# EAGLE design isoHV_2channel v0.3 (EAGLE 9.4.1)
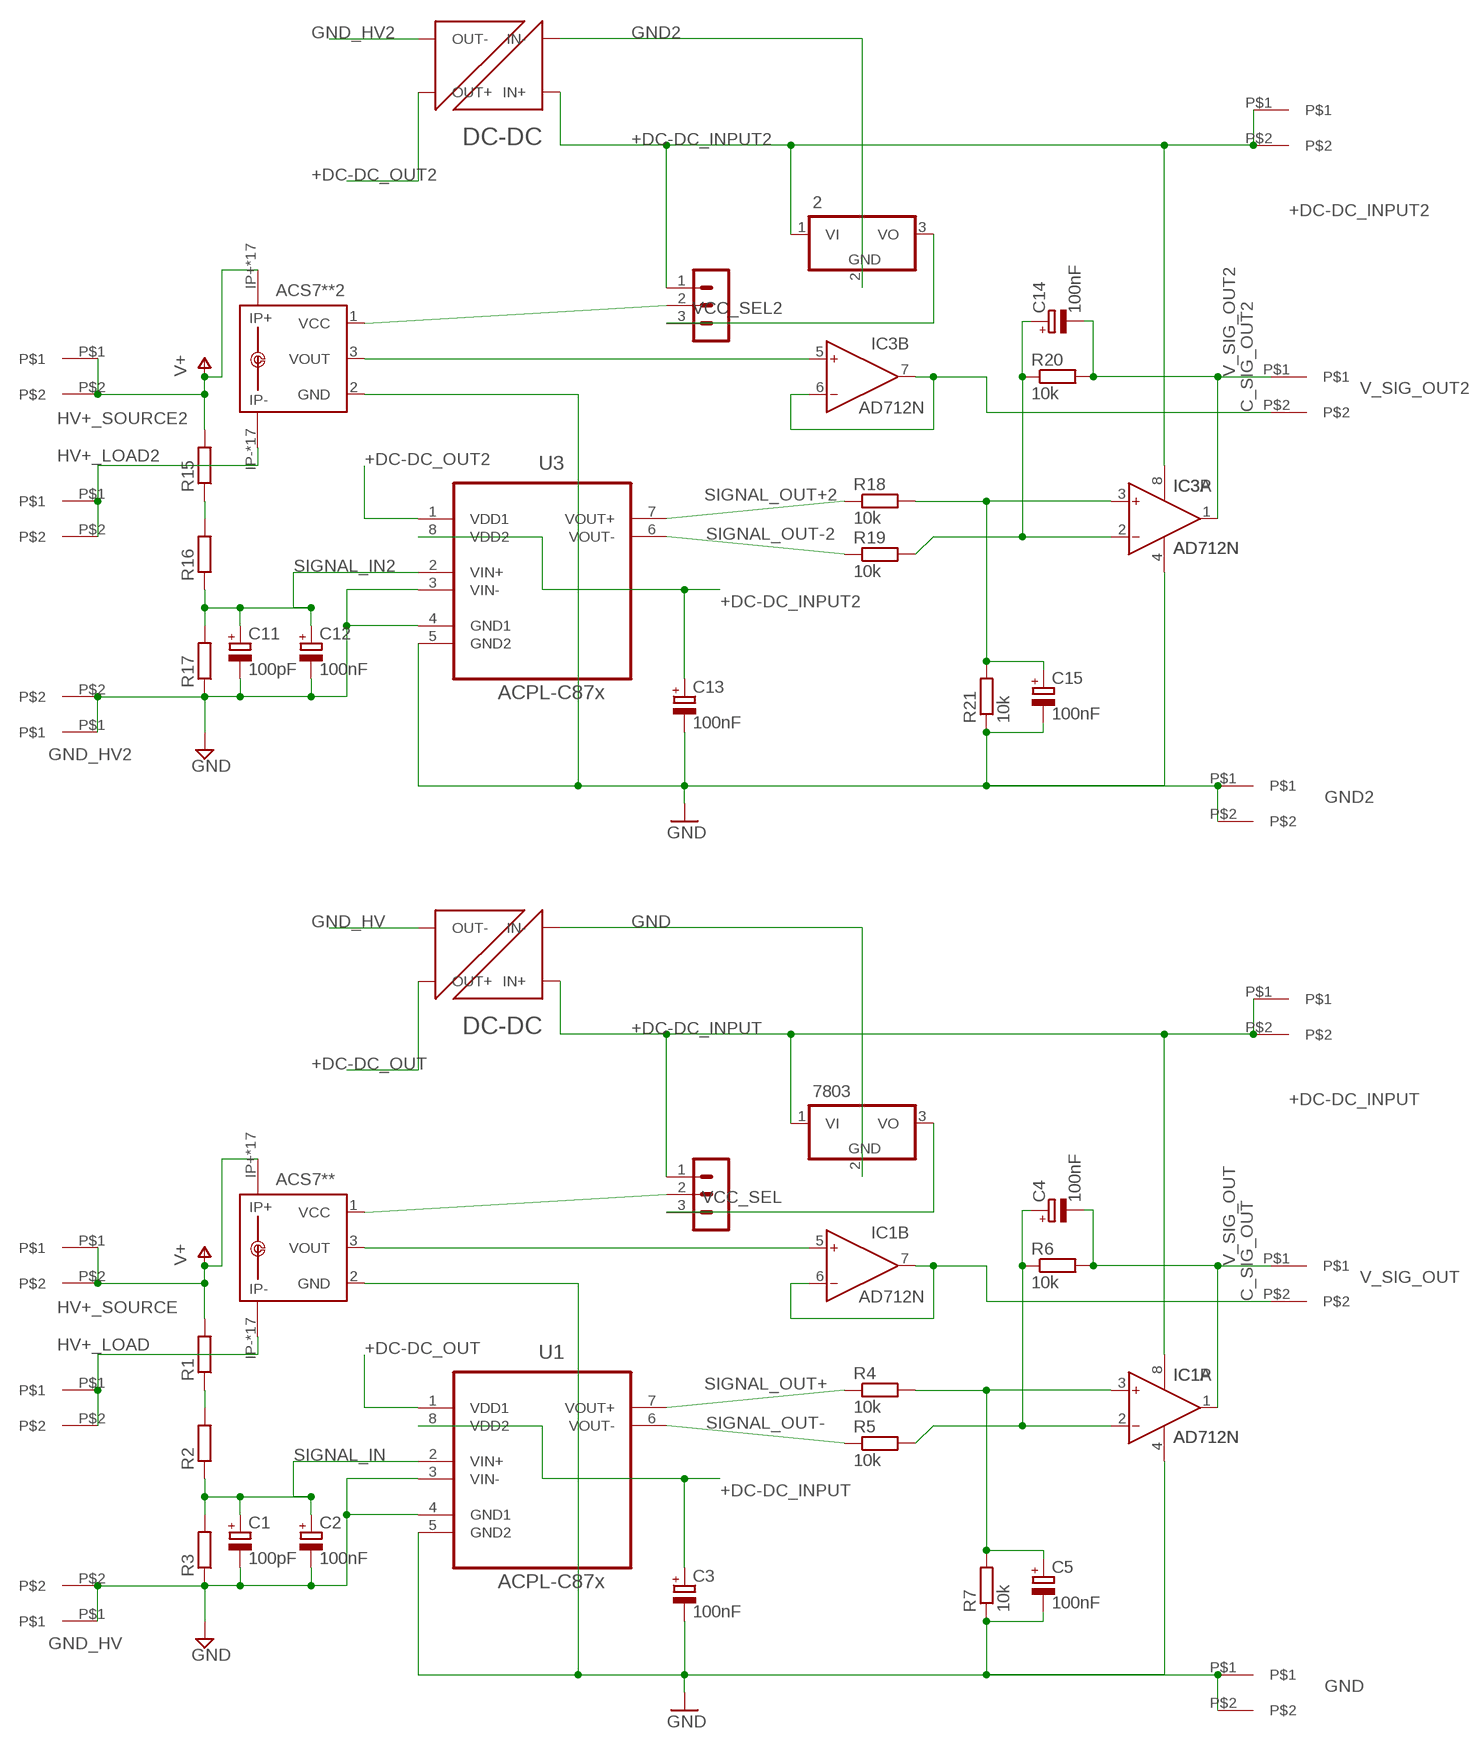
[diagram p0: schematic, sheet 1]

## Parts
2  7805TV  [TO220V]
7803  7805TV  [TO220V]
ACS7**  ACS758KCB-150B-PFF-T  [CB-PFF]
ACS7**2  ACS758KCB-150B-PFF-T  [CB-PFF]
C1  100pF  CPOL-EUB45181A  [B45181A]
C2  100nF  CPOL-EUB45181A  [B45181A]
C3  100nF  CPOL-EUB45181A  [B45181A]
C4  100nF  CPOL-EUB45181A  [B45181A]
C5  100nF  CPOL-EUB45181A  [B45181A]
C11  100pF  CPOL-EUB45181A  [B45181A]
C12  100nF  CPOL-EUB45181A  [B45181A]
C13  100nF  CPOL-EUB45181A  [B45181A]
C14  100nF  CPOL-EUB45181A  [B45181A]
C15  100nF  CPOL-EUB45181A  [B45181A]
IC1  AD712N  [DIL08]
IC3  AD712N  [DIL08]
R1  R-EU_0411/15  [0411/15]
R2  R-EU_0411/15  [0411/15]
R3  R-EU_0411/15  [0411/15]
R4  10k  R-EU_0204/7  [0204/7]
R5  10k  R-EU_0204/7  [0204/7]
R6  10k  R-EU_0204/7  [0204/7]
R7  10k  R-EU_0204/7  [0204/7]
R15  R-EU_0411/15  [0411/15]
R16  R-EU_0411/15  [0411/15]
R17  R-EU_0411/15  [0411/15]
R18  10k  R-EU_0204/7  [0204/7]
R19  10k  R-EU_0204/7  [0204/7]
R20  10k  R-EU_0204/7  [0204/7]
R21  10k  R-EU_0204/7  [0204/7]
U1  ACPL-C87x  ACPL-C79B-000E  [SOIC127P1150X330-8N]
U3  ACPL-C87x  ACPL-C79B-000E  [SOIC127P1150X330-8N]
U$1  7.62MM_TERMINAL_BLOCK  [7.62MM]
U$2  7.62MM_TERMINAL_BLOCK  [7.62MM]
U$3  7.62MM_TERMINAL_BLOCK  [7.62MM]
U$4  7.62MM_TERMINAL_BLOCK  [7.62MM]
U$5  7.62MM_TERMINAL_BLOCK  [7.62MM]
U$6  7.62MM_TERMINAL_BLOCK  [7.62MM]
U$7  NXF1  [NXF1]
U$15  7.62MM_TERMINAL_BLOCK  [7.62MM]
U$16  7.62MM_TERMINAL_BLOCK  [7.62MM]
U$17  7.62MM_TERMINAL_BLOCK  [7.62MM]
U$18  7.62MM_TERMINAL_BLOCK  [7.62MM]
U$19  7.62MM_TERMINAL_BLOCK  [7.62MM]
U$20  7.62MM_TERMINAL_BLOCK  [7.62MM]
U$21  NXF1  [NXF1]
VCC_SEL  MA03-1  [MA03-1]
VCC_SEL2  MA03-1  [MA03-1]

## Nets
+DC-DC_INPUT: 7803.1(VI) C3.+ IC1.8(P:V+) U1.8(VDD2) U$3.P$1 U$3.P$2 U$7.P$3(IN+) VCC_SEL.1
+DC-DC_INPUT2: 2.1(VI) C13.+ IC3.8(P:V+) U3.8(VDD2) U$17.P$1 U$17.P$2 U$21.P$3(IN+) VCC_SEL2.1
+DC-DC_OUT: U1.1(VDD1) U$7.P$8(OUT+)
+DC-DC_OUT2: U3.1(VDD1) U$21.P$8(OUT+)
C_SIG_OUT: IC1.6(B:IN-) IC1.7(B:OUT) U$5.P$2
C_SIG_OUT2: IC3.6(B:IN-) IC3.7(B:OUT) U$19.P$2
GND: 7803.2(GND) ACS7**.2(GND) C3.- C5.- IC1.4(P:V-) R7.1 U1.5(GND2) U$4.P$1 U$4.P$2 U$7.P$1(IN-)
GND2: 2.2(GND) ACS7**2.2(GND) C13.- C15.- IC3.4(P:V-) R21.1 U3.5(GND2) U$18.P$1 U$18.P$2 U$21.P$1(IN-) ; supply symbol labelled GND
GND_HV: C1.- C2.- R3.1 U1.3(VIN-) U1.4(GND1) U$2.P$1 U$2.P$2 U$7.P$7(OUT-) ; supply symbol labelled GND
GND_HV2: C11.- C12.- R17.1 U3.3(VIN-) U3.4(GND1) U$16.P$1 U$16.P$2 U$21.P$7(OUT-) ; supply symbol labelled GND
HV+_LOAD: ACS7**.IP- ACS7**.IP-@2(IP-) ACS7**.IP-@3(IP-) ACS7**.IP-@4(IP-) ACS7**.IP-@5(IP-) ACS7**.IP-@6(IP-) ACS7**.IP-@7(IP-) ACS7**.IP-@8(IP-) ACS7**.IP-@9(IP-) ACS7**.IP-@10(IP-) ACS7**.IP-@11(IP-) ACS7**.IP-@12(IP-) ACS7**.IP-@13(IP-) ACS7**.IP-@14(IP-) ACS7**.IP-@15(IP-) ACS7**.IP-@16(IP-) ACS7**.IP-@17(IP-) U$6.P$1 U$6.P$2
HV+_LOAD2: ACS7**2.IP- ACS7**2.IP-@2(IP-) ACS7**2.IP-@3(IP-) ACS7**2.IP-@4(IP-) ACS7**2.IP-@5(IP-) ACS7**2.IP-@6(IP-) ACS7**2.IP-@7(IP-) ACS7**2.IP-@8(IP-) ACS7**2.IP-@9(IP-) ACS7**2.IP-@10(IP-) ACS7**2.IP-@11(IP-) ACS7**2.IP-@12(IP-) ACS7**2.IP-@13(IP-) ACS7**2.IP-@14(IP-) ACS7**2.IP-@15(IP-) ACS7**2.IP-@16(IP-) ACS7**2.IP-@17(IP-) U$20.P$1 U$20.P$2
HV+_SOURCE: ACS7**.IP+ ACS7**.IP+@2(IP+) ACS7**.IP+@3(IP+) ACS7**.IP+@4(IP+) ACS7**.IP+@5(IP+) ACS7**.IP+@6(IP+) ACS7**.IP+@7(IP+) ACS7**.IP+@8(IP+) ACS7**.IP+@9(IP+) ACS7**.IP+@10(IP+) ACS7**.IP+@11(IP+) ACS7**.IP+@12(IP+) ACS7**.IP+@13(IP+) ACS7**.IP+@14(IP+) ACS7**.IP+@15(IP+) ACS7**.IP+@16(IP+) ACS7**.IP+@17(IP+) R1.2 U$1.P$1 U$1.P$2 ; supply symbol labelled V+
HV+_SOURCE2: ACS7**2.IP+ ACS7**2.IP+@2(IP+) ACS7**2.IP+@3(IP+) ACS7**2.IP+@4(IP+) ACS7**2.IP+@5(IP+) ACS7**2.IP+@6(IP+) ACS7**2.IP+@7(IP+) ACS7**2.IP+@8(IP+) ACS7**2.IP+@9(IP+) ACS7**2.IP+@10(IP+) ACS7**2.IP+@11(IP+) ACS7**2.IP+@12(IP+) ACS7**2.IP+@13(IP+) ACS7**2.IP+@14(IP+) ACS7**2.IP+@15(IP+) ACS7**2.IP+@16(IP+) ACS7**2.IP+@17(IP+) R15.2 U$15.P$1 U$15.P$2 ; supply symbol labelled V+
N$1: C5.+ IC1.3(A:IN+) R4.2 R7.2
N$2: R1.1 R2.2
N$3: ACS7**.1(VCC) VCC_SEL.2
N$5: C4.+ IC1.2(A:IN-) R5.2 R6.1
N$6: ACS7**.3(VOUT) IC1.5(B:IN+)
N$7: 7803.3(VO) VCC_SEL.3
N$132: R15.1 R16.2
N$142: C15.+ IC3.3(A:IN+) R18.2 R21.2
N$152: C14.+ IC3.2(A:IN-) R19.2 R20.1
N$162: ACS7**2.1(VCC) VCC_SEL2.2
N$172: ACS7**2.3(VOUT) IC3.5(B:IN+)
N$182: 2.3(VO) VCC_SEL2.3
SIGNAL_IN: C1.+ C2.+ R2.1 R3.2 U1.2(VIN+)
SIGNAL_IN2: C11.+ C12.+ R16.1 R17.2 U3.2(VIN+)
SIGNAL_OUT+: R4.1 U1.7(VOUT+)
SIGNAL_OUT+2: R18.1 U3.7(VOUT+)
SIGNAL_OUT-: R5.1 U1.6(VOUT-)
SIGNAL_OUT-2: R19.1 U3.6(VOUT-)
V_SIG_OUT: C4.- IC1.1(A:OUT) R6.2 U$5.P$1
V_SIG_OUT2: C14.- IC3.1(A:OUT) R20.2 U$19.P$1

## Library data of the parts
2 7803 = linear:78*: Positive VOLTAGE REGULATOR Source: http://cache.national.com/ds/LM/LM78L05.pdf http://www.fairchildsemi.com/ds/LM/LM7805.pdf
ACS7** ACS7**2 = allegro:ACS758*: Thermally Enhanced, Fully Integrated, Hall Effect-Based Linear Current Sensor with 100 micro Ohm Current Conductor display layer 49 Reference in BRD and place VIAs on circles Source: http://www.allegromicro.com/en/Products/Part_Numbers/0758/0758.pdf; MPN: ACS7**; OC_FARNELL: 1718995; OC_NEWARK: 04R7129
C1-C5 C11-C15 = rcl:CPOL-EU: POLARIZED CAPACITOR, European symbol; SPICEPREFIX: C
IC1 IC3 = analog-devices:AD712: Dual Precision, Low Cost, High Speed BiFET Op Amp Source: http://www.analog.com/static/imported-files/data_sheets/AD712.pdf; MF: ALTERA CORPORATION; MPN: AD712JNZ; OC_FARNELL: 9604898; OC_NEWARK: 59K4554
R1-R7 R15-R21 = rcl:R-EU_: RESISTOR, European symbol; SPICEPREFIX: R
U1 U3 = Avago_By_element14_Batch_1:ACPL-C79B-000E: Precision Miniature Isolation Amplifiers; DESCRIPTION: Precision Miniature Isolation Amplifiers; MPN: ACPL-C79B-000E; OC_FARNELL: 1854253; OC_NEWARK: 74R5803; PACKAGE: SOIC-8; SUPPLIER: AVAGO TECHNOLOGIES
U$1-U$6 U$15-U$20 = 7.62mm terminal block:7.62MM_TERMINAL_BLOCK
U$7 U$21 = NXF1:NXF1
VCC_SEL VCC_SEL2 = con-lstb:MA03-1: PIN HEADER; OC_FARNELL: unknown; OC_NEWARK: unknown

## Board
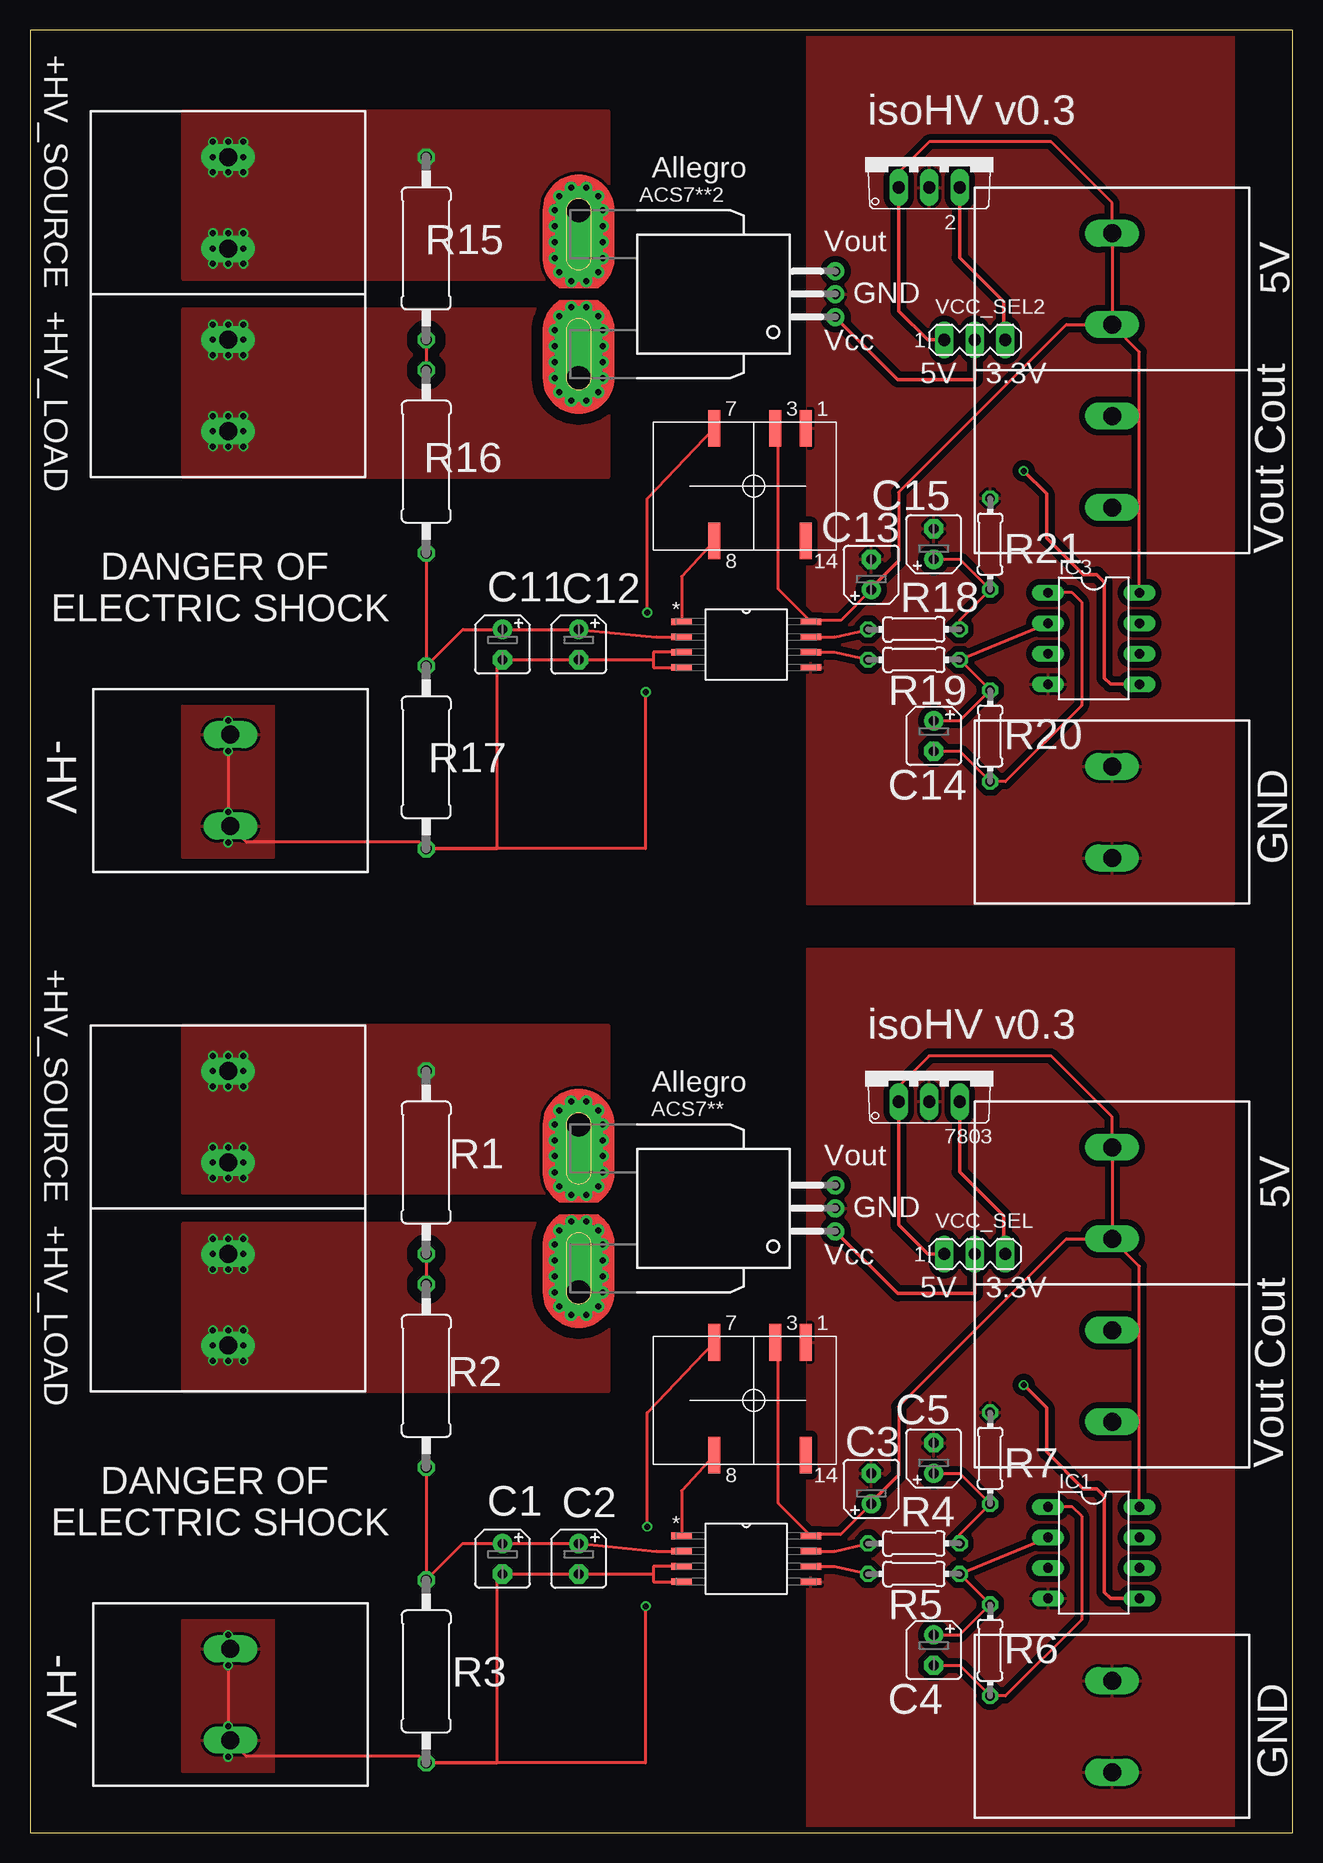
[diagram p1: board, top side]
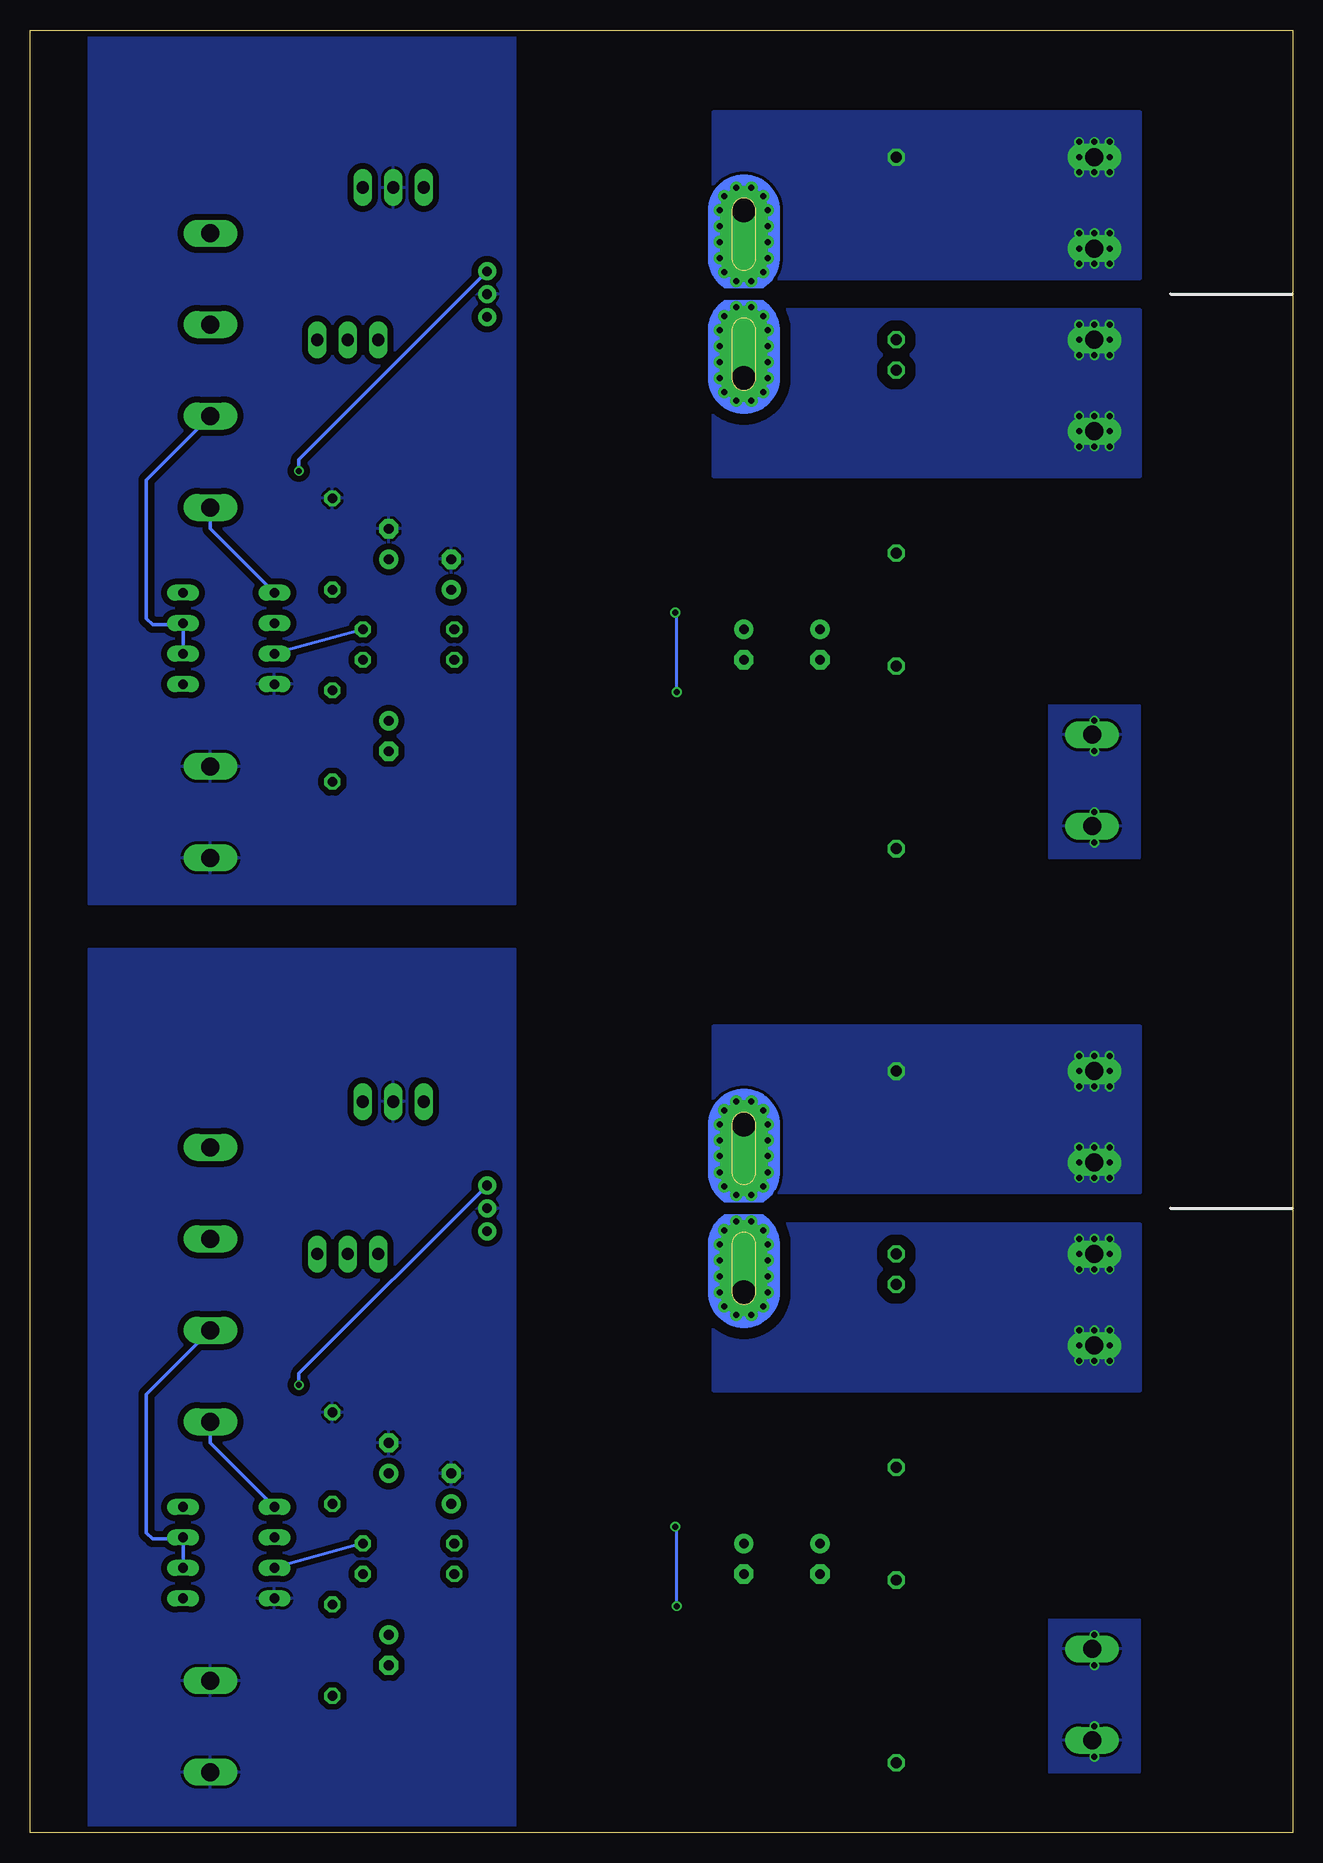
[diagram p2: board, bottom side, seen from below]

Size 105.21 x 150.29 mm. Coordinates in mm from the lower left corner, seen from the top.
Outline: 0,150.29 0,0 105.21,0 105.21,150.29 0,150.29
Copper layers (1*16): Top 0.07111875mm / dielectric 1.45776875mm / Bottom 0.07111875mm
Design rules "jlcpcb *": minimum track width 6mil, minimum drill 12mil, track to track 10mil, track to pad 10mil, pad to pad 10mil, via to via 10mil, smd to smd 0mil, copper to edge 10mil, drill to drill 10mil, minimum pad ring 10mil, minimum via ring 6mil, stop-mask expansion 2mil, vias tented up to drill 25mil, thermal gap 10mil

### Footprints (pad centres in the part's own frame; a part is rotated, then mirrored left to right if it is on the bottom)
TO220V = drill 1.016 long: 1 -2.54,-2.54; 2 0,-2.54; 3 2.54,-2.54
CB-PFF = drill 0.8 pad 1.5: 1 -1.91,-21.4; 2 0,-21.4; 3 1.91,-21.4 | drill 2 pad 4 offset: IP+ 7,0; IP- -7,0 | drill 0.5 pad 0.9: IP+@2 8.89,0.635; IP+@3 8.89,-0.635; IP+@4 8.175,-1.625; IP+@5 7,-2; IP+@6 5.675,-2; IP+@7 4.35,-2; IP+@8 3,-2; IP+@9 1.825,-1.625; IP+@10 1.1,-0.625; IP+@11 1.1,0.625; IP+@12 1.825,1.625; IP+@13 3,2; IP+@14 4.35,2; IP+@15 5.675,2; IP+@16 7,2; IP+@17 8.175,1.625; IP-@2 -8.89,0.635; IP-@3 -8.89,-0.635; IP-@4 -8.175,-1.625; IP-@5 -7,-2; IP-@6 -5.675,-2; IP-@7 -4.325,-2; IP-@8 -3,-2; IP-@9 -1.825,-1.625; IP-@10 -1.1,-0.625; IP-@11 -1.1,0.625; IP-@12 -1.825,1.625; IP-@13 -3,2; IP-@14 -4.325,2; IP-@15 -5.675,2; IP-@16 -7,2; IP-@17 -8.175,1.625
B45181A = drill 0.813 pad 1.6: + -1.27,0 | drill 0.813 pad 1.6 octagon: - 1.27,0
DIL08 = drill 0.813 long: 1 -3.81,-3.81; 2 -1.27,-3.81; 3 1.27,-3.81; 4 3.81,-3.81; 5 3.81,3.81; 6 1.27,3.81; 7 -1.27,3.81; 8 -3.81,3.81
0411/15 = drill 0.914 octagon: 1 -7.62,0; 2 7.62,0
0204/7 = drill 0.813 octagon: 1 -3.81,0; 2 3.81,0
SOIC127P1150X330-8N = smd 1.702 x 0.559: 1 -5.385,1.905; 2 -5.385,0.635; 3 -5.385,-0.635; 4 -5.385,-1.905; 5 5.385,-1.905; 6 5.385,-0.635; 7 5.385,0.635; 8 5.385,1.905
7.62MM = drill 1.5 long: P$1 0,-3.81; P$2 0,3.81
NXF1 = smd 0.991 x 3.048: P$1 -4.318,-4.826; P$3 -1.778,-4.826; P$7 3.302,-4.826; P$8 3.302,4.572; P$14 -4.318,4.572
MA03-1 = drill 1.016 long: 1 -2.54,0; 2 0,0; 3 2.54,0

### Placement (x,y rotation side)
2  74.93,139.7 0 top
7803  74.93,63.5 0 top
ACS7**  45.72,52.07 90 top
ACS7**2  45.72,128.27 90 top
C1  39.37,22.86 270 top
C2  45.72,22.86 270 top
C3  70.1,28.7 90 top
C4  75.31,15.24 270 top
C5  75.31,31.24 90 top
C11  39.37,99.06 270 top
C12  45.72,99.06 270 top
C13  70.1,104.9 90 top
C14  75.31,91.44 270 top
C15  75.31,107.44 90 top
IC1  88.65,23.37 270 top
IC3  88.65,99.57 270 top
R1  33.02,55.88 90 top
R2  33.02,38.1 90 top
R3  33.02,13.46 90 top
R4  73.66,24.13 0 top
R5  73.66,21.59 0 top
R6  80.01,15.24 270 top
R7  80.01,31.24 270 top
R15  33.02,132.08 90 top
R16  33.02,114.3 90 top
R17  33.02,89.66 90 top
R18  73.66,100.33 0 top
R19  73.66,97.79 0 top
R20  80.01,91.44 270 top
R21  80.01,107.44 270 top
U1  59.69,22.86 0 top
U3  59.69,99.06 0 top
U$1  16.51,59.69 180 top
U$2  16.7,11.54 0 top
U$3  90.17,53.34 0 top
U$4  90.17,8.89 180 top
U$5  90.17,38.1 0 top
U$6  16.51,44.45 0 top
U$7  60.33,36.07 180 top
U$15  16.51,135.89 180 top
U$16  16.7,87.74 0 top
U$17  90.17,129.54 0 top
U$18  90.17,85.09 180 top
U$19  90.17,114.3 0 top
U$20  16.51,120.65 0 top
U$21  60.33,112.27 180 top
VCC_SEL  78.74,48.26 0 top
VCC_SEL2  78.74,124.46 0 top

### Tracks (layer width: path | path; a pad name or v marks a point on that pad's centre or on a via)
+DC-DC_INPUT
  Top 0.254: IC1.8 92.46,47.24 U$3.P$1 | U$3.P$1 U$3.P$2 90.17,59.69 85.09,64.77 74.93,64.77 72.39,62.23 7803.1 | 72.39,30.73 72.39,35.56 86.36,49.53 U$3.P$1 | C3.+ 67.55,24.88 65.08,24.88 U1.8 62.36,27.48 62.36,40.59 U$7.P$3
  Top 0.305: 7803.1 72.39,50.67 74.8,48.26 VCC_SEL.1 | 72.39,30.73 72.39,29.84 70.1,27.56 C3.+
+DC-DC_INPUT2
  Top 0.254: IC3.8 92.46,123.44 U$17.P$1 | U$17.P$1 U$17.P$2 90.17,135.89 85.09,140.97 74.93,140.97 72.39,138.43 2.1 | 72.39,106.93 72.39,111.76 86.36,125.73 U$17.P$1 | C13.+ 67.55,101.08 65.08,101.08 U3.8 62.36,103.68 62.36,116.79 U$21.P$3
  Top 0.305: 2.1 72.39,126.87 74.8,124.46 VCC_SEL2.1 | 72.39,106.93 72.39,106.05 70.1,103.76 C13.+
+DC-DC_OUT
  Top 0.254: U1.1 54.3,28.54 U$7.P$8
+DC-DC_OUT2
  Top 0.254: U3.1 54.3,104.74 U$21.P$8
C_SIG_OUT
  Bottom 0.305: U$5.P$2 95.5,36.58 95.5,25.02 95,24.51 92.58,24.51 IC1.7 IC1.6
C_SIG_OUT2
  Bottom 0.305: U$19.P$2 95.5,112.78 95.5,101.22 95,100.71 92.58,100.71 IC3.7 IC3.6
GND
  pour Bottom (isolate 0.508): 100.33,73.66 100.33,0 64.77,0 64.77,73.66
  pour Top (isolate 0.508): 64.77,73.66 64.77,0 100.33,0 100.33,73.66
GND2
  pour Bottom (isolate 0.508): 100.33,149.86 100.33,77.47 64.77,77.47 64.77,149.86
  pour Top (isolate 0.508): 64.77,151.13 64.77,77.47 100.33,77.47 100.33,151.13
GND_HV  (via drill 0.5)
  Top 0.254: U1.3 51.94,22.23 51.94,21.59 | 51.94,21.59 51.94,20.95 U1.4 | U$2.P$2 16.7,14.16 v16.51,13.97 v16.51,8.89 16.7,8.7 U$2.P$1 18.04,6.39 32.47,6.39 R3.1 | R3.1 38.9,5.84 38.9,21.12 C1.- C2.- 51.94,21.59 | R3.1 51.31,5.84 v51.31,18.9 | v51.44,25.53 51.44,35.02 U$7.P$7
  Bottom 0.254: v51.31,18.9 51.31,25.4 v51.44,25.53
  other vias: 16.51,16.51 16.51,6.35
  pour Top: 12.7,17.78 20.32,17.78 20.32,5.08 12.7,5.08
  pour Bottom: 12.7,17.78 20.32,17.78 20.32,5.08 12.7,5.08
GND_HV2  (via drill 0.5)
  Top 0.254: U3.3 51.94,98.42 51.94,97.79 | 51.94,97.79 51.94,97.16 U3.4 | U$16.P$2 16.7,90.36 v16.51,90.17 v16.51,85.09 16.7,84.9 U$16.P$1 18.04,82.59 32.47,82.59 R17.1 | R17.1 38.9,82.04 38.9,97.32 C11.- C12.- 51.94,97.79 | R17.1 51.31,82.04 v51.31,95.1 | v51.44,101.73 51.44,111.22 U$21.P$7
  Bottom 0.254: v51.31,95.1 51.31,101.6 v51.44,101.73
  other vias: 16.51,92.71 16.51,82.55
  pour Top: 12.7,93.98 20.32,93.98 20.32,81.28 12.7,81.28
  pour Bottom: 12.7,93.98 20.32,93.98 20.32,81.28 12.7,81.28
HV+_LOAD  (via drill 0.5)
  other vias: 16.51,46.99 15.24,49.53 16.51,49.53 17.78,49.53 17.78,48.26 17.78,46.99 15.24,46.99 15.24,48.26 17.78,41.91 17.78,40.64 17.78,39.37 16.51,39.37 15.24,39.37 15.24,40.64 15.24,41.91 16.51,41.91
  pour Bottom (isolate 0.889, no thermals): 48.26,50.8 12.7,50.8 12.7,36.83 48.26,36.83
  pour Top (isolate 0.889, no thermals): 48.26,50.8 12.7,50.8 12.7,36.83 48.26,36.83
HV+_LOAD2  (via drill 0.5)
  other vias: 16.51,123.19 15.24,125.73 16.51,125.73 17.78,125.73 17.78,124.46 17.78,123.19 15.24,123.19 15.24,124.46 17.78,118.11 17.78,116.84 17.78,115.57 16.51,115.57 15.24,115.57 15.24,116.84 15.24,118.11 16.51,118.11
  pour Bottom (isolate 0.889, no thermals): 48.26,127 12.7,127 12.7,113.03 48.26,113.03
  pour Top (isolate 0.889, no thermals): 48.26,127 12.7,127 12.7,113.03 48.26,113.03
HV+_SOURCE  (via drill 0.5)
  other vias: 15.24,57.15 16.51,57.15 17.78,57.15 17.78,55.88 17.78,54.61 16.51,54.61 15.24,54.61 15.24,55.88 16.51,62.23 17.78,62.23 17.78,63.5 17.78,64.77 16.51,64.77 15.24,64.77 15.24,63.5 15.24,62.23
  pour Top (no thermals): 46.99,48.26 48.26,49.53 48.26,48.26
  pour Bottom (no thermals): 12.7,53.34 48.26,53.34 48.26,67.31 12.7,67.31
  pour Top (no thermals): 12.7,53.34 48.26,53.34 48.26,67.31 12.7,67.31
HV+_SOURCE2  (via drill 0.5)
  other vias: 15.24,133.35 16.51,133.35 17.78,133.35 17.78,132.08 17.78,130.81 16.51,130.81 15.24,130.81 15.24,132.08 16.51,138.43 17.78,138.43 17.78,139.7 17.78,140.97 16.51,140.97 15.24,140.97 15.24,139.7 15.24,138.43
  pour Top (no thermals): 46.99,124.46 48.26,125.73 48.26,124.46
  pour Bottom (no thermals): 12.7,129.54 48.26,129.54 48.26,143.51 12.7,143.51
  pour Top (no thermals): 12.7,129.54 48.26,129.54 48.26,143.51 12.7,143.51
N$1
  Top 0.254: R4.2 77.47,24.89 R7.2 77.47,29.97 C5.+
  Bottom 0.254: R4.2 IC1.3
N$2
  Top 0.254: R1.1 R2.2
N$3
  Top 0.305: VCC_SEL.2 78.74,44.96 72.32,44.96 ACS7**.1
N$5
  Top 0.254: IC1.2 R5.2 R6.1 77.47,16.51 C4.+
N$6  (via drill 0.5)
  Top 0.305: v82.8,37.34 84.71,35.43 84.71,31.75 87.76,28.7 88.9,28.7 89.53,28.07 89.53,20.07 90.04,19.56 IC1.5
  Bottom 0.305: v82.8,37.34 82.8,38.3 ACS7**.3
N$7
  Top 0.305: 7803.3 77.47,55.12 81.15,51.44 81.15,48.39 VCC_SEL.3
N$132
  Top 0.254: R15.1 R16.2
N$142
  Top 0.254: R18.2 77.47,101.09 R21.2 77.47,106.17 C15.+
  Bottom 0.254: R18.2 IC3.3
N$152
  Top 0.254: IC3.2 R19.2 R20.1 77.47,92.71 C14.+
N$162
  Top 0.305: VCC_SEL2.2 78.74,121.16 72.32,121.16 ACS7**2.1
N$172  (via drill 0.5)
  Top 0.305: v82.8,113.54 84.71,111.63 84.71,107.95 87.76,104.9 88.9,104.9 89.53,104.27 89.53,96.27 90.04,95.76 IC3.5
  Bottom 0.305: v82.8,113.54 82.8,114.5 ACS7**2.3
N$182
  Top 0.305: 2.3 77.47,131.32 81.15,127.64 81.15,124.59 VCC_SEL2.3
SIGNAL_IN
  Top 0.254: R2.1 R3.2 36.07,24.13 C1.+ C2.+ 52.2,23.5 U1.2
SIGNAL_IN2
  Top 0.254: R16.1 R17.2 36.07,100.33 C11.+ C12.+ 52.2,99.69 U3.2
SIGNAL_OUT+
  Top 0.254: U1.7 67.06,23.5 R4.1
SIGNAL_OUT+2
  Top 0.254: U3.7 67.06,99.69 R18.1
SIGNAL_OUT-
  Top 0.254: U1.6 67.06,22.23 R5.1
SIGNAL_OUT-2
  Top 0.254: U3.6 67.06,98.42 R19.1
V_SIG_OUT
  Top 0.254: C4.- 77.47,13.97 R6.2 81.28,11.43 87.63,17.78 87.63,26.42 86.87,27.18 IC1.1
  Bottom 0.305: U$5.P$1 90.17,32.51 IC1.1
V_SIG_OUT2
  Top 0.254: C14.- 77.47,90.17 R20.2 81.28,87.63 87.63,93.98 87.63,102.62 86.87,103.38 IC3.1
  Bottom 0.305: U$19.P$1 90.17,108.71 IC3.1

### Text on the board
tNames: +HV_SOURCE | isoHV v0.3 | Allegro | Vout | GND | 5V | +HV_LOAD | Vcc | 5V | 3.3V | Cout | Vout | DANGER OF / ELECTRIC SHOCK | -HV | GND | +HV_SOURCE | isoHV v0.3 | Allegro | Vout | 5V | +HV_LOAD | GND | Vcc | 5V | 3.3V | Cout | Vout | DANGER OF / ELECTRIC SHOCK | -HV | GND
